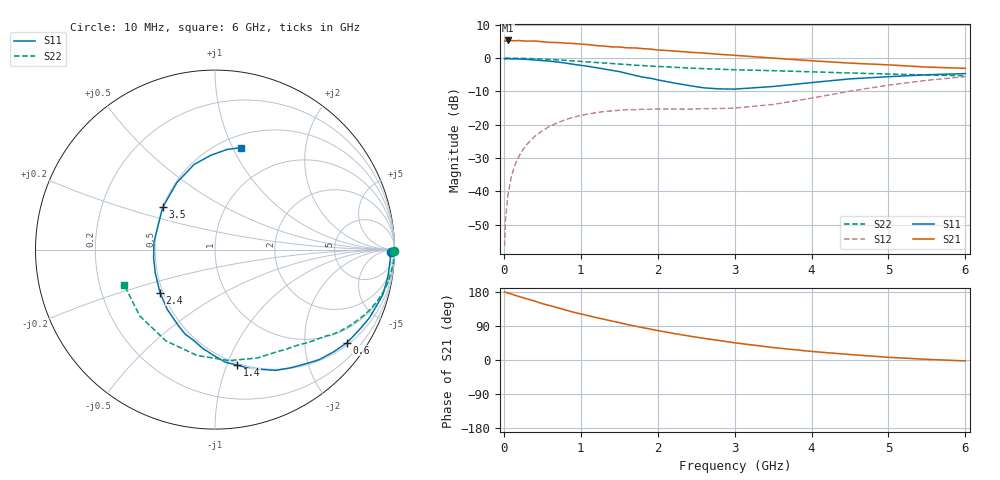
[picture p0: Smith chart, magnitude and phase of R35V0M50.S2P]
! SIEMENS Small Signal Semiconductors
! BFR181
! Si NPN RF Bipolar Junction Transistor in SOT23
! VCE = 5 V  IC = 0.5 mA
! Common Emitter S-Parameters:  May  1996
# GHz  S  MA  R  50
!  f  S11  S21  S12  S22
! GHz  MAG  ANG  MAG  ANG  MAG  ANG  MAG  ANG
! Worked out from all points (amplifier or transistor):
!   36 points, 10 MHz to 6 GHz, reference 50 ohm
!   highest |S21| = 5.3 dB at 50 MHz (marker M1)
!   |S21| within 3 dB of that: start of sweep to 2.099 GHz
!   unconditionally stable (mu >= 1): 2.368 GHz to 3.941 GHz
!   at 250 MHz: K = 0.12, MSG = 16.3 dB, |S12| = -27.5 dB
!   at 1.4 GHz: K = 0.60, MSG = 9.6 dB, |S12| = -15.8 dB
!   at 6 GHz: K = 0.92, MSG = 1.2 dB, |S12| = -5.6 dB
!   S11 on the Smith chart (normalised r, x): 10 MHz: 70, -40; 600 MHz: 0.56, -3.07; 1.4 GHz: 0.48, -1.09; 2.4 GHz: 0.48, -0.27; 3.5 GHz: 0.50, +0.28; 6 GHz: 0.62, +1.08
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0.01  0.9787 -0.7  1.818 179.8  0.0015 96.3  0.9992 -0.3
0.02  0.9704 -1.0  1.791 178.8  0.0035 87.9  0.9982 -0.6
0.05  0.9787 -2.8  1.844 177.0  0.0084 87.9  0.9986 -1.4
0.1  0.9761 -5.7  1.832 174.2  0.0172 86.2  0.9999 -2.8
0.15  0.975 -8.8  1.827 170.3  0.0258 83.9  0.9958 -4.3
0.2  0.9707 -11.7  1.842 167.4  0.0341 81.3  0.9927 -5.6
0.3  0.9582 -17.7  1.803 161.2  0.0509 77.3  0.9865 -8.4
0.4  0.9411 -23.7  1.81 155.7  0.0667 73.4  0.9786 -11.2
0.5  0.9191 -29.3  1.765 148.7  0.0811 69.7  0.9676 -13.9
0.6  0.9002 -35.1  1.725 143.5  0.0952 65.8  0.9548 -16.4
0.9  0.8103 -51.9  1.661 126.4  0.1293 55.5  0.909 -23.5
1.1  0.7532 -63.3  1.596 116.8  0.1452 49.8  0.8763 -27.7
1.4  0.6563 -79.0  1.477 102.9  0.1613 42.5  0.8311 -33.3
1.7  0.5533 -97.3  1.425 89.7  0.1685 37.9  0.7841 -37.8
2.2  0.4263 -128.6  1.284 70.4  0.1722 34.3  0.7311 -45.2
2.4  0.3887 -142.0  1.23 63.5  0.1716 35.0  0.71 -48.1
3  0.3428 172.7  1.104 45.4  0.1779 40.4  0.6688 -57.8
3.5  0.3752 140.8  1.001 32.9  0.2016 47.3  0.6481 -68.8
4.5  0.4886 103.8  0.842 14.4  0.3192 50.4  0.5984 -99.6
5  0.5266 92.4  0.793 7.1  0.3935 45.4  0.5774 -118.3
5.5  0.5628 82.9  0.734 1.8  0.4647 38.0  0.559 -138.5
6  0.5862 75.6  0.703 -2.5  0.5274 29.2  0.5427 -158.6
